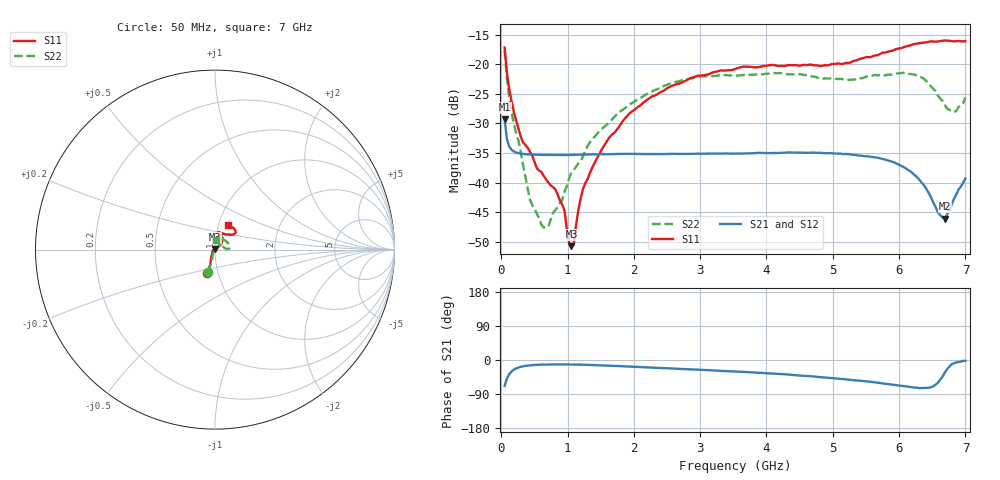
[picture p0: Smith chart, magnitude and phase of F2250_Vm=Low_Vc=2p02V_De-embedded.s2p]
! Integrated Device Technology
! Corporate Headquarters
! 6024 Silver Creek Valley Road
! San Jose, CA 95138  USA
! Phone:  1-408-284-8200
! Toll Free:  1-800-223-1366
! Webpage:  http://www.idt.com/
! Timing and RF Division
! 515 Groton Road, Suite 102
! Westford, MA 01886-6024
! Device:  F2250
! Description: Voltage Variable RF Attenuator
! Frequency:  50.0 -  6000.00 MHz
! Package:  3x3 mm Thin QFN Plastic Package: 16 pin
! Ports:  2 RF, 3 DC
!  Pin  1  = GND
!  Pin  2  = NC
!  Pin  3  = RF1  = Port 1
!  Pin  4  = NC
!  Pin  5  = GND
!  Pin  6  = GND
!  Pin  7  = GND
!  Pin  8  = GND
!  Pin  9  = NC
!  Pin 10  = RF2  = Port 2
!  Pin 11  = NC
!  Pin 12  = GND
!  Pin 13  = GND
!  Pin 14  = VCNTRL
!  Pin 15  = VDD
!  Pin 16  = VMODE
! Vcntrl:  2.020 Volts
! Vmode:  +0.000 Volts
! Vdd:  +3.30  Volts
! Current:  1.183 mA
! Data:  The device was measured on a the F2250 evaluation board which has
!  individual transmission lines to the RF pins.  Data was collected
!  using a calibrated network analyzer.  The evaluation board was
!  de-embedded using a TRL calibration technique.
!  The reference plane is the edge of the package pin.
! Misc:  SN 10
!  Action Tracker AT0258
! Date Measured:  2014-11-26
! Date:  2015-10-15  MJV
! Note:
!  Integrated Device Technology supplies this data as a sample of measured
!  data at the package pin for this product.  Your particular data for this
!  product may vary.
!  Data was taken at 25 degrees C.
!  Integrated Device Technology reserves the right to change this data at anytime.
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# GHz S dB R 50
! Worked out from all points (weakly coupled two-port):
!   201 points, 50 MHz to 7 GHz, reference 50 ohm
!   highest |S21| = -29.29 dB at 50 MHz (marker M1); lowest = -46.1 dB at 6.687 GHz (marker M2)
!   lowest |S11| = -50.7 dB at 1.058 GHz (marker M3), VSWR 1.01, Z = 49.8 + j0.245 ohm
!   |S11| at or under -10 dB: start of sweep to end of sweep
!   |S22| runs from -47.6 to -17.8 dB; largest |S21 - S12| = 5.8e-05
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0.05  -17.18 -108.6  -29.29 -68.4  -29.29 -68.4  -17.75 -108.7
0.08475  -21.44 -107.4  -32.67 -49.1  -32.68 -49.1  -22.42 -104.5
0.1195  -24.19 -111.7  -33.89 -37.5  -33.89 -37.5  -25.71 -107.5
0.29325  -32.20 -127.6  -35.08 -18.1  -35.08 -18.1  -34.73 -115.5
0.43225  -34.74 -144.5  -35.23 -14.1  -35.23 -14.1  -42.90 -145.3
0.606  -38.19 -161.0  -35.30 -12.2  -35.29 -12.2  -47.07 160.7
0.71025  -39.98 -168.4  -35.31 -11.8  -35.32 -11.8  -47.41 122.4
0.91875  -43.64 158.1  -35.33 -11.7  -35.33 -11.7  -42.90 83.3
1.023  -50.10 143.8  -35.32 -11.8  -35.32 -11.8  -39.19 71.4
1.05775  -50.70 122.4  -35.31 -11.8  -35.32 -11.8  -38.30 68.8
1.0925  -50.48 88.9  -35.30 -11.9  -35.30 -11.9  -37.84 64.3
1.162  -44.62 56.2  -35.29 -12.2  -35.28 -12.1  -36.72 55.5
1.2315  -41.09 44.1  -35.26 -12.4  -35.26 -12.4  -35.59 49.5
1.6485  -32.11 41.8  -35.18 -15.1  -35.18 -15.1  -29.56 46.7
2.37825  -24.88 47.3  -35.15 -20.9  -35.15 -20.9  -24.08 47.6
3.525  -20.81 72.4  -35.09 -30.4  -35.09 -30.4  -21.93 70.0
4.7065  -20.17 72.3  -34.91 -43.5  -34.91 -43.5  -22.10 69.5
5.85325  -17.82 40.4  -36.31 -64.0  -36.31 -64.1  -21.74 18.0
6.33975  -16.40 41.0  -39.98 -74.0  -39.98 -74.0  -22.22 3.9
6.68725  -15.99 48.8  -46.06 -33.6  -46.05 -33.1  -26.85 24.1
6.861  -16.12 55.1  -42.01 -6.3  -41.96 -6.3  -27.91 58.6
7  -16.12 63.2  -39.28 -2.1  -39.23 -2.2  -25.61 86.9
